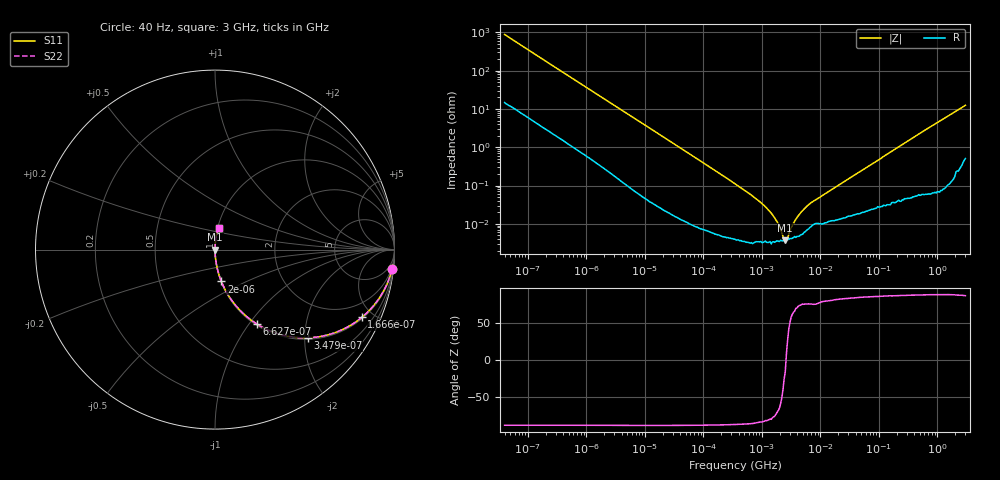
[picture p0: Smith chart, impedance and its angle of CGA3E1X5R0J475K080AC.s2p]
! S-parameter Generated by TDK Corporation
! Copyright(C) 2015 TDK Corporation.
! All Rights Reserved.
! TDK P/N: CGA3E1X5R0J475K080AC (Multilayer Ceramic Chip Capacitors)
! Property: C=4.7uF
! Size(LxWxT): 1.6x0.8x0.8mm, 0.063x0.031x0.031inches
! Model Type: s2p (Touchstone File Format Version 1.0)
! Frequency: DC=Yes Start=0.00004MHz Stop=3000MHz 396points Log-sweep
! Note: This model was converted from impedance.
! Model Generated on Jun. 23, 2015
! Hash(MD5):
! Port Assignments:
!  1 ---| |--- 2
! Applicable Conditions:
!  Temperature = 25 degC
!  DC Bias Voltage = 0 V
!  Small Signal Operation
! Terms and conditions regarding TDK Simulation Models
! (1)This simulation model is being provided solely for informational purposes. Please refer to the specifications of the products in terms of detailed characteristics of such products.
! (2)In no event shall TDK Corporation of any of its subsidiaries be liable for any loss or damage arising, directly or indirectly,
!  From any information contained in this simulation model, including, but not limited to loss or damages arising from any inaccuracies, omissions or errors in connection with such information.
! (3)Any and all copyrights on this simulation model are owned by TDK Corporation.
!  Duplication or redistribution of this simulation model without prior written permission from TDK Corporation is prohibited.
! (4)This simulation model is subject to any modification or change without any prior notice.
! (5)Neither TDK Corporation nor any of its subsidiaries shall make any warranty, express or implied,
!  Including but not limited to the correctness, implied warranties of merchantability and fitness for a particular purpose with respect to this simulation models.
! (6)The use of this simulation model shall be deemed to have consented to the terms and conditions hereof.
# MHz S MA R 50
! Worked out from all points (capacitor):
!   395 points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, 40 Hz to 3 GHz, reference 50 ohm
!   read as one part in series: C = 4.49 uF near 41.88 Hz
!   lowest |Z| = 3.71 mohm at 2.506 MHz (marker M1)
!   series resonance near 2.581 MHz, so ESL is about 850 pH
!   S11 on the Smith chart (normalised r, x): 40 Hz: 1, -18; 166.6 Hz: 1.07, -4.30; 347.9 Hz: 1.03, -2.07; 662.7 Hz: 1.02, -1.09; 2 kHz: 1.01, -0.37; 3 GHz: 1.01, +0.25
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4e-05  0.9919 -6.4  0.1118 82.6  0.1118 82.6  0.9919 -6.4
9.158711e-05  0.9647 -14.3  0.2478 74.7  0.2478 74.7  0.9647 -14.3
0.0001665986  0.9011 -24.8  0.4189 64.3  0.4189 64.3  0.9011 -24.8
0.0003479132  0.7137 -43.5  0.6887 45.5  0.6887 45.5  0.7137 -43.5
0.000662667  0.477 -60.6  0.8712 28.5  0.8712 28.5  0.477 -60.6
0.000834128  0.3974 -65.7  0.9113 23.4  0.9113 23.4  0.3974 -65.7
0.001262176  0.2774 -73.0  0.9564 16.1  0.9564 16.1  0.2774 -73.0
0.001999837  0.1811 -78.7  0.9807 10.4  0.9807 10.4  0.1811 -78.7
0.005020464  0.07469 -85.0  0.9962 4.3  0.9962 4.3  0.07469 -85.0
0.01739424  0.02205 -88.0  0.9995 1.3  0.9995 1.3  0.02205 -88.0
0.3464102  0.001117 -87.9  1 0.1  1 0.1  0.001117 -87.9
0.6301264  0.0005918 -86.9  1 0.0  1 0.0  0.0005918 -86.9
1.094655  0.0002983 -83.5  1 0.0  1 0.0  0.0002983 -83.5
1.442786  0.0001895 -81.0  1 0.0  1 0.0  0.0001895 -81.0
1.901634  9.788e-05 -69.0  1 0.0  1 0.0  9.788e-05 -69.0
2.506407  3.708e-05 -15.7  1 0.0  1 0.0  3.708e-05 -15.7
3.459106  0.0001036 65.0  1 -0.0  1 -0.0  0.0001036 65.0
4.773931  0.0002096 75.6  0.9999 -0.0  0.9999 -0.0  0.0002096 75.6
7.22376  0.0003724 76.0  0.9999 -0.0  0.9999 -0.0  0.0003724 76.0
150.6385  0.00718 87.1  0.9997 -0.4  0.9997 -0.4  0.00718 87.1
906.6656  0.04069 86.7  0.9985 -2.3  0.9985 -2.3  0.04069 86.7
3000  0.1237 80.6  0.9873 -7.1  0.9873 -7.1  0.1237 80.6
